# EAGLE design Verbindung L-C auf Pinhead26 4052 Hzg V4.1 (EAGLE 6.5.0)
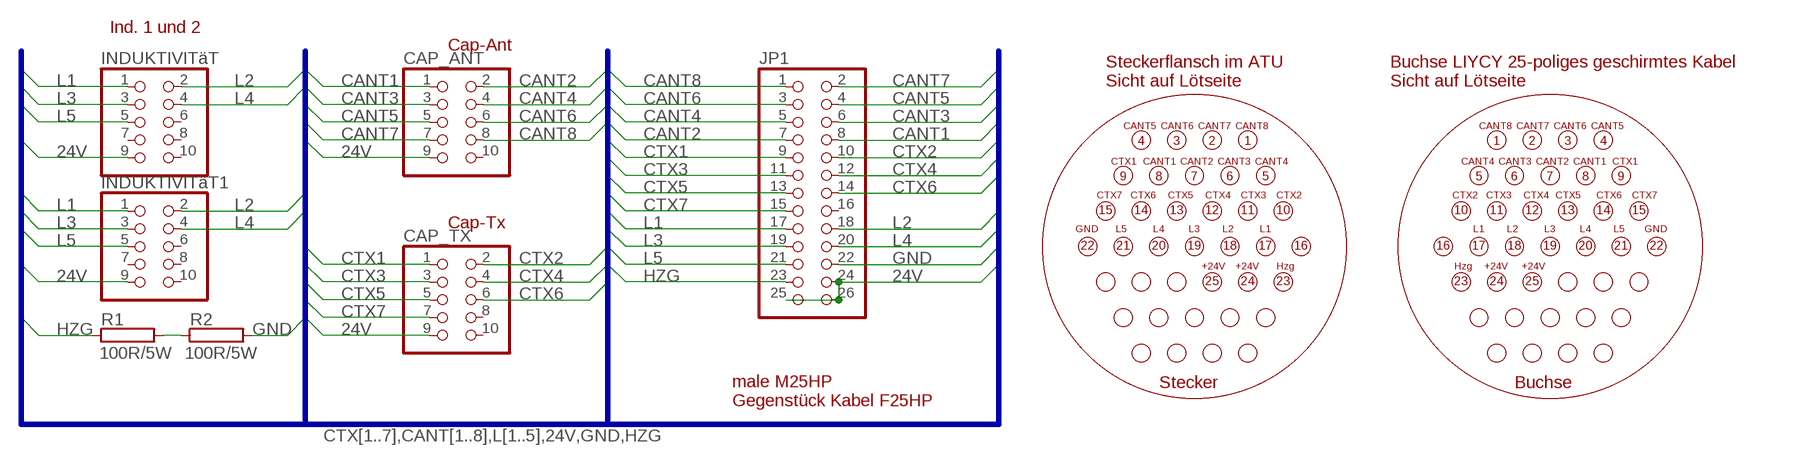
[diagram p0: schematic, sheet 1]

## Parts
CAP_ANT  PINHD-2X5  [2X05]
CAP_TX  PINHD-2X5  [2X05]
INDUKTIVITäT  PINHD-2X5  [2X05]
INDUKTIVITäT1  PINHD-2X5  [2X05]
JP1  PINHD-2X13  [2X13]
R1  100R/5W  RKH208-8  [KH208-8]
R2  100R/5W  RKH208-8  [KH208-8]

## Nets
24V: CAP_ANT.9 CAP_TX.9 INDUKTIVITäT1.9 INDUKTIVITäT.9 JP1.24 JP1.25 JP1.26
CANT1: CAP_ANT.1 JP1.8
CANT2: CAP_ANT.2 JP1.7
CANT3: CAP_ANT.3 JP1.6
CANT4: CAP_ANT.4 JP1.5
CANT5: CAP_ANT.5 JP1.4
CANT6: CAP_ANT.6 JP1.3
CANT7: CAP_ANT.7 JP1.2
CANT8: CAP_ANT.8 JP1.1
CTX1: CAP_TX.1 JP1.9
CTX2: CAP_TX.2 JP1.10
CTX3: CAP_TX.3 JP1.11
CTX4: CAP_TX.4 JP1.12
CTX5: CAP_TX.5 JP1.13
CTX6: CAP_TX.6 JP1.14
CTX7: CAP_TX.7 JP1.15
GND: JP1.22 R2.2
HZG: JP1.23 R1.1
L1: INDUKTIVITäT1.1 INDUKTIVITäT.1 JP1.17
L2: INDUKTIVITäT1.2 INDUKTIVITäT.2 JP1.18
L3: INDUKTIVITäT1.3 INDUKTIVITäT.3 JP1.19
L4: INDUKTIVITäT1.4 INDUKTIVITäT.4 JP1.20
L5: INDUKTIVITäT1.5 INDUKTIVITäT.5 JP1.21
N$1: R1.2 R2.1
Unconnected: CAP_ANT.10 CAP_TX.8 CAP_TX.10 INDUKTIVITäT1.6 INDUKTIVITäT1.7 INDUKTIVITäT1.8 INDUKTIVITäT1.10 INDUKTIVITäT.6 INDUKTIVITäT.7 INDUKTIVITäT.8 INDUKTIVITäT.10 JP1.16

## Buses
CTX[1..7],CANT[1..8],L[1..5],24V,GND,HZG

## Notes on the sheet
- Ind. 1 und 2
- Cap-Ant
- Steckerflansch im ATU 
  Sicht auf Lötseite
- Buchse LIYCY 25-poliges geschirmtes Kabel 
  Sicht auf Lötseite
- CANT5 | CANT6 | CANT7 | CANT8 | CANT8 | CANT7 | CANT6 | CANT5
- 4 | 3 | 2 | 1 | 1 | 2 | 3 | 4
- CANT1 | CANT2 | CANT3 | CANT4 | CANT4 | CANT3 | CANT2 | CANT1
- CTX1 | CTX1
- 9 | 8 | 7 | 6 | 5 | 5 | 6 | 7 | 8 | 9
- CTX7 | CTX6 | CTX5 | CTX4 | CTX3 | CTX2 | CTX2 | CTX3 | CTX4 | CTX5 | CTX6 | CTX7
- 15 | 14 | 13 | 12 | 11 | 10 | 10 | 11 | 12 | 13 | 14 | 15
- Cap-Tx
- GND | L5 | L4 | L3 | L2 | L1 | L1 | L2 | L3 | L4 | L5 | GND
- 22 | 21 | 20 | 19 | 18 | 17 | 16 | 16 | 17 | 18 | 19 | 20 | 21 | 22
- +24V | +24V | Hzg | Hzg | +24V | +24V
- 25 | 24 | 23 | 23 | 24 | 25
- Stecker | Buchse
- male M25HP 
  Gegenstück Kabel F25HP

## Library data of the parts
CAP_ANT CAP_TX INDUKTIVITäT INDUKTIVITäT1 = pinhead+:PINHD-2X5: PIN HEADER
JP1 = pinhead+:PINHD-2X13: PIN HEADER
R1 R2 = resistor-power:R: Power Resitor; OC_FARNELL: unknown; OC_NEWARK: unknown

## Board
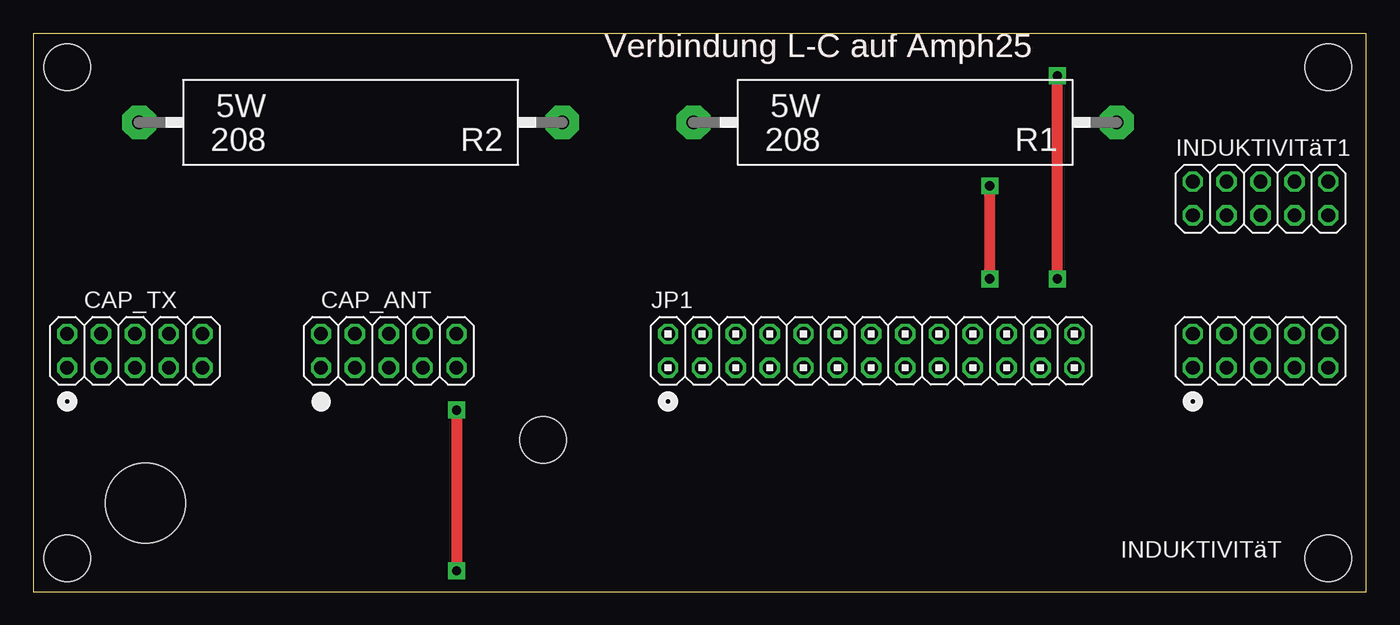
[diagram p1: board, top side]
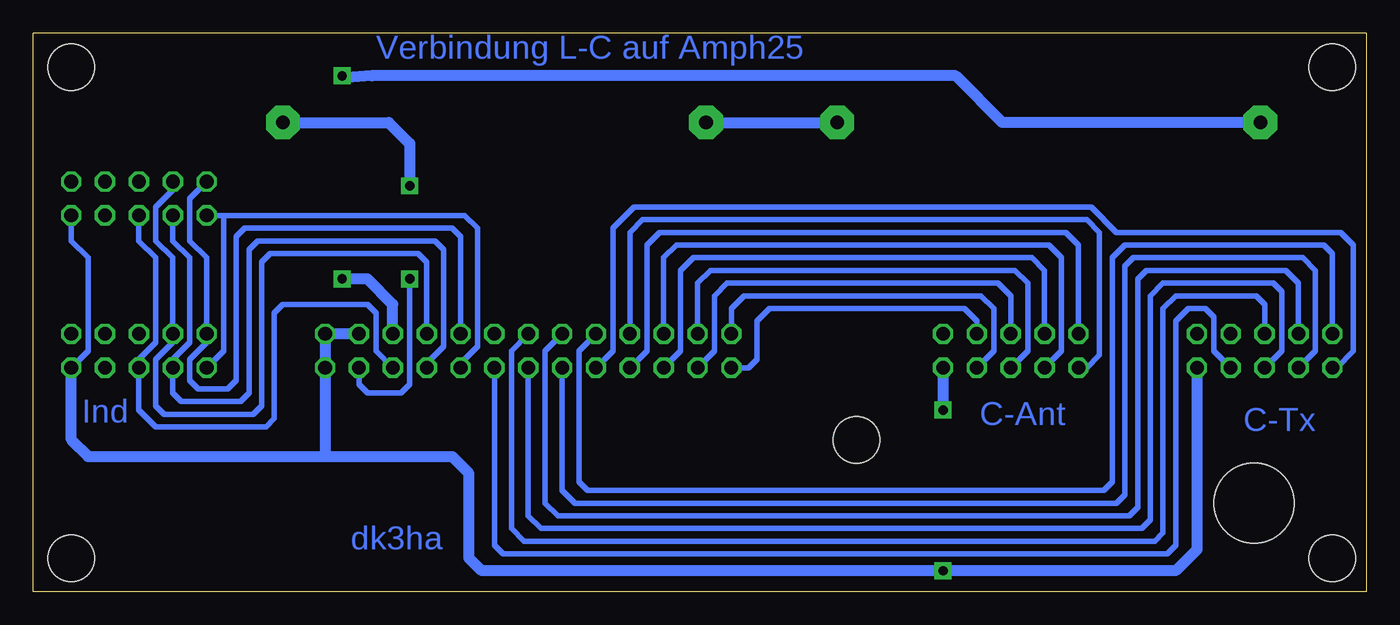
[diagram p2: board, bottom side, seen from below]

Size 100 x 41.91 mm. Coordinates in mm from the lower left corner, seen from the top.
Outline: 0,41.91 0,0 100,0 100,41.91 0,41.91
Copper layers (1*16): Top 0.035mm / dielectric 1.5mm / Bottom 0.035mm
Design rules "default *": minimum track width 10mil, minimum drill 24mil, track to track 8mil, track to pad 8mil, pad to pad 8mil, via to via 8mil, smd to smd 8mil, copper to edge 0mil, drill to drill 8mil, minimum pad ring 10mil, minimum via ring 8mil, stop-mask expansion 4mil, vias tented up to drill 0mil, thermal gap 10mil
Holes 3.5 mm at 2.54,2.52 97.16,2.52 97.16,39.35 2.54,39.35 38.26,11.41
Holes 6 mm at 8.41,6.65

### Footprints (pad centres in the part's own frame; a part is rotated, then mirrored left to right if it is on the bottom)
2X05 = drill 1.016 octagon: 1 -5.08,-1.27; 2 -5.08,1.27; 3 -2.54,-1.27; 4 -2.54,1.27; 5 0,-1.27; 6 0,1.27; 7 2.54,-1.27; 8 2.54,1.27; 9 5.08,-1.27; 10 5.08,1.27
2X13 = drill 1.016 octagon: 1 -15.24,-1.27; 2 -15.24,1.27; 3 -12.7,-1.27; 4 -12.7,1.27; 5 -10.16,-1.27; 6 -10.16,1.27; 7 -7.62,-1.27; 8 -7.62,1.27; 9 -5.08,-1.27; 10 -5.08,1.27; 11 -2.54,-1.27; 12 -2.54,1.27; 13 0,-1.27; 14 0,1.27; 15 2.54,-1.27; 16 2.54,1.27; 17 5.08,-1.27; 18 5.08,1.27; 19 7.62,-1.27; 20 7.62,1.27; 21 10.16,-1.27; 22 10.16,1.27; 23 12.7,-1.27; 24 12.7,1.27; 25 15.24,-1.27; 26 15.24,1.27
KH208-8 = drill 1.016 pad 2.54 octagon: 1 -15.875,0; 2 15.875,0

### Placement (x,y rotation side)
CAP_ANT  26.67,18.08 0 top
CAP_TX  7.62,18.08 0 top
INDUKTIVITäT  92.08,18.08 0 top
INDUKTIVITäT1  92.08,29.51 0 top
JP1  62.87,18.08 0 top
R1  65.41,35.22 180 top
R2  23.81,35.22 180 top

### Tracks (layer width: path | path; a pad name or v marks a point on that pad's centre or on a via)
24V  (via drill 0.7 pad 1.27)
  Top 0.813: v31.75,13.63 v31.75,1.57
  Bottom 0.406: INDUKTIVITäT1.9 97.16,26.33 95.89,25.06 95.89,18.08 INDUKTIVITäT.9
  Bottom 0.813: JP1.24 JP1.26 JP1.25 78.11,10.14 | CAP_TX.9 12.7,3.15 14.29,1.57 v31.75,1.57 66.36,1.57 67.31,2.52 67.31,8.87 68.58,10.14 78.11,10.14 | INDUKTIVITäT.9 97.16,11.41 95.89,10.14 78.11,10.14 | CAP_ANT.9 v31.75,13.63
CANT1
  Bottom 0.406: CAP_ANT.1 20.95,16.81 20,17.76 20,26.97 20.95,27.92 54.29,27.92 55.24,26.97 JP1.8
CANT2
  Bottom 0.406: CAP_ANT.2 21.59,26.02 22.54,26.97 53.02,26.97 53.98,26.02 53.98,18.08 JP1.7
CANT3
  Bottom 0.406: CAP_ANT.3 22.86,18.08 22.86,25.06 23.81,26.02 51.75,26.02 52.7,25.06 JP1.6
CANT4
  Bottom 0.406: CAP_ANT.4 24.13,24.11 25.08,25.06 50.48,25.06 51.44,24.11 51.44,18.08 JP1.5
CANT5
  Bottom 0.406: CAP_ANT.5 25.4,18.08 25.4,23.16 26.35,24.11 49.21,24.11 50.16,23.16 JP1.4
CANT6
  Bottom 0.406: CAP_ANT.6 26.67,22.21 27.62,23.16 47.94,23.16 48.9,22.21 48.9,18.08 JP1.3
CANT7
  Bottom 0.406: CAP_ANT.7 27.94,18.08 27.94,21.25 28.89,22.21 46.67,22.21 47.62,21.25 JP1.2
CANT8
  Bottom 0.406: CAP_ANT.8 29.21,20.3 30.16,21.25 44.77,21.25 45.72,20.3 45.72,17.44 46.35,16.81 JP1.1
CTX1
  Bottom 0.406: CAP_TX.1 2.22,16.81 0.95,18.08 0.95,26.02 1.91,26.97 18.73,26.97 20.64,28.87 54.93,28.87 56.52,27.29 56.52,18.08 JP1.9
CTX2
  Bottom 0.406: CAP_TX.2 2.54,25.38 3.17,26.02 18.1,26.02 19.05,25.06 19.05,8.24 19.68,7.6 58.42,7.6 59.05,8.24 59.05,18.08 JP1.10
CTX3
  Bottom 0.406: CAP_TX.3 3.81,18.08 3.81,24.11 4.76,25.06 17.46,25.06 18.1,24.43 18.1,7.28 18.73,6.65 59.37,6.65 60.33,7.6 JP1.11
CTX4
  Bottom 0.406: CAP_TX.4 5.08,23.16 6.03,24.11 16.51,24.11 17.14,23.48 17.14,6.33 17.78,5.7 60.64,5.7 61.59,6.65 61.59,18.08 JP1.12
CTX5
  Bottom 0.406: CAP_TX.5 6.35,18.08 6.35,22.52 6.99,23.16 15.24,23.16 16.19,22.21 16.19,5.38 16.83,4.74 61.91,4.74 62.87,5.7 JP1.13
CTX6
  Bottom 0.406: CAP_TX.6 7.62,21.57 8.26,22.21 14.29,22.21 15.24,21.25 15.24,4.43 15.88,3.79 63.18,3.79 64.14,4.74 64.14,18.08 JP1.14
CTX7
  Bottom 0.406: CAP_TX.7 11.43,18.08 11.43,20.62 12.06,21.25 13.34,21.25 14.29,20.3 14.29,3.47 14.92,2.84 64.77,2.84 65.41,3.47 JP1.15
GND  (via drill 0.7 pad 1.27)
  Top 0.813: v76.83,23.48 v76.83,38.71
  Bottom 0.813: JP1.22 73.03,21.57 74.93,23.48 v76.83,23.48 | v76.83,38.71 76.99,38.56 74.61,38.71 30.8,38.71 27.3,35.22 R2.2
HZG  (via drill 0.7 pad 1.27)
  Top 0.813: v71.75,23.48 v71.75,30.46
  Bottom 0.406: JP1.23 75.56,15.54 74.93,14.9 72.39,14.9 71.75,15.54 v71.75,23.48
  Bottom 0.813: R1.1 73.34,35.22 71.75,33.63 v71.75,30.46
L1
  Bottom 0.406: 85.72,28.24 85.72,18.08 INDUKTIVITäT.1 | JP1.17 67.94,17.12 66.67,18.39 66.67,27.29 67.63,28.24 85.72,28.24 | 85.72,28.24 INDUKTIVITäT1.1
L2
  Bottom 0.406: INDUKTIVITäT1.2 88.27,29.51 88.27,26.33 87,25.06 INDUKTIVITäT.2 87,18.71 88.27,17.44 88.27,15.86 87.63,15.22 85.41,15.22 84.77,15.86 84.77,26.65 84.14,27.29 68.58,27.29 67.94,26.65 JP1.18
L3
  Bottom 0.406: INDUKTIVITäT1.3 89.53,26.33 88.27,25.06 88.27,18.71 89.53,17.44 INDUKTIVITäT.3 89.53,14.9 88.9,14.27 84.45,14.27 83.82,14.9 83.82,25.7 83.19,26.33 69.85,26.33 69.22,25.7 69.22,18.39 70.48,17.12 JP1.19
L4
  Bottom 0.406: INDUKTIVITäT1.4 89.53,30.14 90.81,28.87 90.81,26.33 89.53,25.06 INDUKTIVITäT.4 89.53,18.71 90.81,17.44 90.81,13.95 90.17,13.32 83.5,13.32 82.87,13.95 82.87,24.75 82.23,25.38 71.12,25.38 70.48,24.75 JP1.20
L5
  Bottom 0.406: INDUKTIVITäT1.5 92.08,26.33 90.81,25.06 90.81,18.71 92.08,17.44 INDUKTIVITäT.5 92.08,13.63 90.81,12.36 82.55,12.36 81.92,13 81.92,20.93 81.28,21.57 74.93,21.57 74.3,20.93 74.3,18.08 JP1.21
N$1
  Bottom 0.813: R1.2 R2.1

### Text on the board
Top: Verbindung L-C auf Amph25
Bottom: Verbindung L-C auf Amph25 | C-Ant | Ind | C-Tx | dk3ha
tPlace: Verbindung L-C auf Amph25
